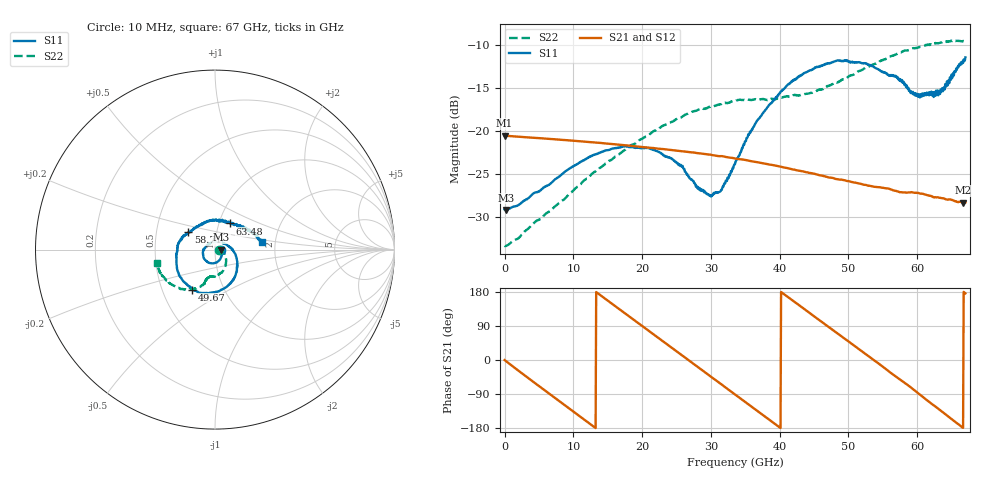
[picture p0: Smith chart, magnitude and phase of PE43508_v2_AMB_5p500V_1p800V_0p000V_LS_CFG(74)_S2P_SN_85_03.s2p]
!Keysight Technologies,N5227A,US51270237,A.10.43.00
!Date: Wednesday, August 22, 2018 17:14:21
!Correction: S11(Full 2 Port(1,3))
!S31(Full 2 Port(1,3))
!S13(Full 2 Port(1,3))
!S33(Full 2 Port(1,3))
!S2P File: Measurements: S11, S31, S13, S33:
# Hz S  dB  R 50
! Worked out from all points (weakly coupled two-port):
!   801 points, 10 MHz to 67 GHz, reference 50 ohm
!   highest |S21| = -20.55 dB at 10 MHz (marker M1); lowest = -28.3 dB at 66.67 GHz (marker M2)
!   lowest |S11| = -29.2 dB at 261.2 MHz (marker M3), VSWR 1.07, Z = 53.6 - j0.0933 ohm
!   |S11| at or under -10 dB: start of sweep to end of sweep
!   |S22| runs from -33.4 to -9.5 dB; largest |S21 - S12| = 0.00049
!   S11 on the Smith chart (normalised r, x): 10 MHz: 1.07, -0.00; 49.67 GHz: 0.71, -0.34; 58.71 GHz: 0.73, +0.14; 63.48 GHz: 1.13, +0.34; 67 GHz: 1.71, +0.15
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1e7  -29.14 -0.7  -20.55 -0.2  -20.55 -0.2  -33.33 -0.5
2.612125e8  -29.19 -1.4  -20.58 -3.8  -20.59 -3.8  -33.35 1.0
5.871625e9  -26.46 -36.2  -20.90 -80.5  -20.90 -80.5  -29.68 -1.4
1.123082e10  -23.51 -73.2  -21.23 -152.7  -21.24 -152.7  -26.01 -17.9
1.74274e10  -21.82 -114.4  -21.67 124.3  -21.67 124.3  -22.25 -38.1
2.236791e10  -22.43 -149.9  -22.08 58.2  -22.07 58.2  -19.80 -54.7
2.571741e10  -24.09 177.6  -22.38 13.6  -22.37 13.6  -18.44 -65.7
2.990429e10  -27.46 106.0  -22.76 -42.7  -22.76 -42.7  -17.24 -79.0
3.14953e10  -26.86 68.1  -22.94 -63.7  -22.94 -63.8  -16.92 -84.4
3.3505e10  -23.87 29.0  -23.20 -91.0  -23.21 -91.0  -16.53 -90.3
3.55147e10  -20.48 1.0  -23.47 -117.9  -23.48 -117.9  -16.38 -94.3
3.836178e10  -17.15 -27.4  -23.89 -155.9  -23.90 -155.8  -16.40 -99.8
4.137632e10  -14.58 -53.5  -24.37 163.7  -24.37 163.8  -16.05 -102.6
4.472582e10  -12.91 -80.8  -24.93 119.1  -24.92 119.2  -15.60 -104.9
4.966634e10  -11.82 -119.5  -25.80 53.3  -25.79 53.3  -13.88 -108.2
5.276462e10  -12.31 -145.9  -26.33 11.9  -26.31 11.8  -12.58 -114.2
5.586291e10  -13.62 -178.6  -26.70 -29.9  -26.70 -30.3  -11.46 -123.6
5.870999e10  -15.01 147.1  -27.15 -67.4  -27.16 -67.7  -10.65 -133.1
6.130585e10  -15.88 101.7  -27.42 -104.6  -27.43 -104.9  -10.06 -143.2
6.348302e10  -15.45 59.7  -27.79 -134.7  -27.84 -135.3  -9.75 -152.2
6.666505e10  -12.15 13.6  -28.32 -179.1  -28.39 -179.1  -9.58 -165.1
6.7e10  -11.50 8.6  -28.31 175.9  -28.40 175.8  -9.54 -166.8
